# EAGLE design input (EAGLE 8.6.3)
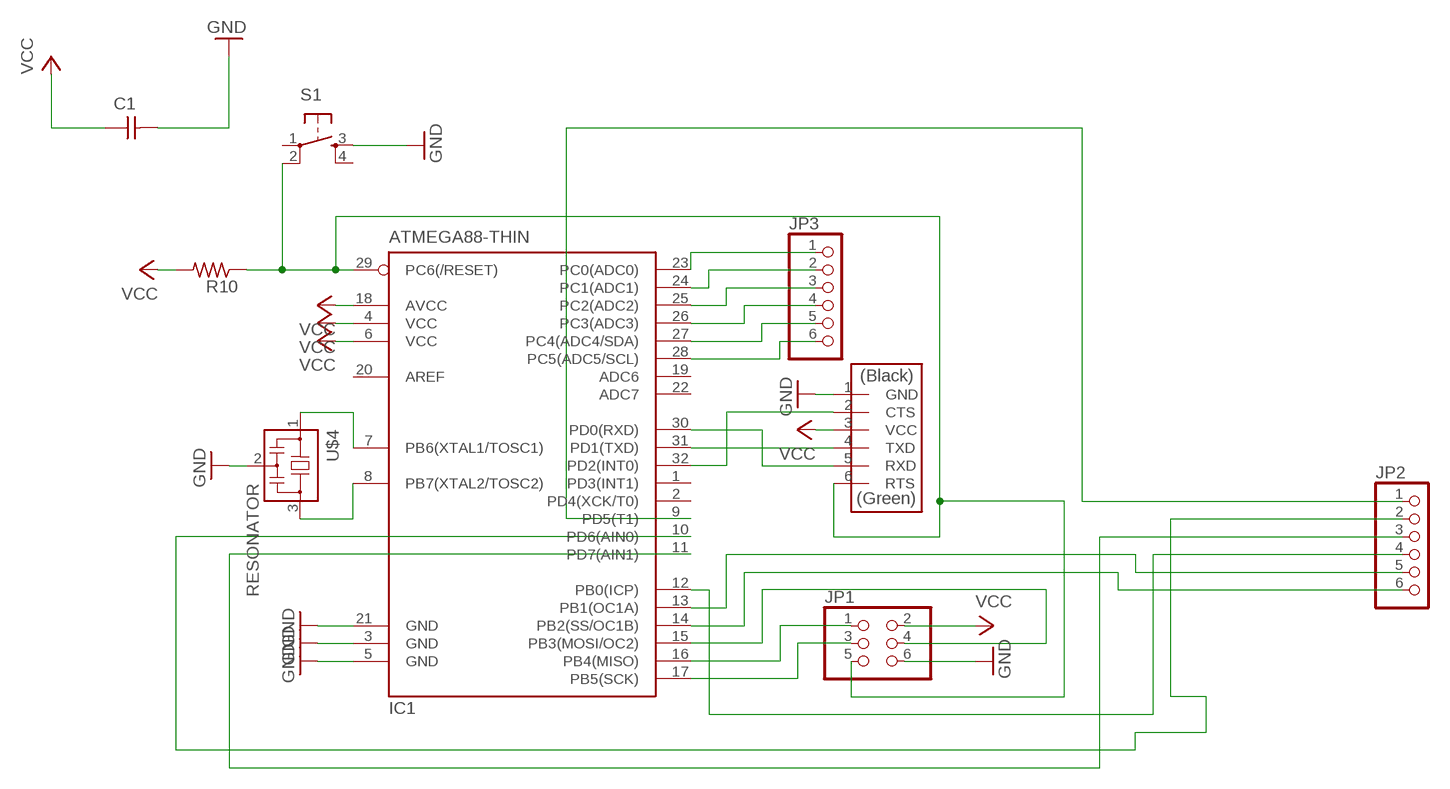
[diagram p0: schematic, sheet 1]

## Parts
C1  CAP-UNPOLARIZEDFAB  [C1206FAB]
IC1  ATMEGA88-THIN  [TQFP32-08THIN]
JP1  PINHD-2X3-SMD  [2X03SMD]
JP2  PINHD-1X6  [1X06]
JP3  PINHD-1X6  [1X06]
R10  RES-US1206FAB  [R1206FAB]
S1  6MM_SWITCH6MM_SWITCH  [6MM_SWITCH]
U$4  RESONATOR  [EFOBM]
U$5  FTDI-SMD-HEADER  [1X06SMD]

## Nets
GND: C1.2 IC1.3(GND) IC1.5(GND) IC1.21(GND) JP1.6 S1.3(S) U$4.2 U$5.1(GND)
N$1: IC1.7(PB6(XTAL1/TOSC1)) U$4.1
N$2: IC1.8(PB7(XTAL2/TOSC2)) U$4.3
N$3: IC1.29(PC6(/RESET)) JP1.5 R10.1 S1.2(P1) U$5.6(RTS)
N$4: IC1.15(PB3(MOSI/OC2)) JP1.4
N$5: IC1.31(PD1(TXD)) U$5.4(TXD)
N$6: IC1.16(PB4(MISO)) JP1.1
N$7: IC1.28(PC5(ADC5/SCL)) JP3.6
N$8: IC1.17(PB5(SCK)) JP1.3
N$9: IC1.30(PD0(RXD)) U$5.5(RXD)
N$10: IC1.32(PD2(INT0)) U$5.2(CTS)
N$11: IC1.27(PC4(ADC4/SDA)) JP3.5
N$12: IC1.26(PC3(ADC3)) JP3.4
N$13: IC1.25(PC2(ADC2)) JP3.3
N$14: IC1.24(PC1(ADC1)) JP3.2
N$15: IC1.23(PC0(ADC0)) JP3.1
N$16: IC1.14(PB2(SS/OC1B)) JP2.6
N$17: IC1.13(PB1(OC1A)) JP2.5
N$18: IC1.12(PB0(ICP)) JP2.4
N$19: IC1.11(PD7(AIN1)) JP2.3
N$20: IC1.10(PD6(AIN0)) JP2.2
N$21: IC1.9(PD5(T1)) JP2.1
VCC: C1.1 IC1.4(VCC) IC1.6(VCC) IC1.18(AVCC) JP1.2 R10.2 U$5.3(VCC)
Unconnected: IC1.1(PD3(INT1)) IC1.2(PD4(XCK/T0)) IC1.19(ADC6) IC1.20(AREF) IC1.22(ADC7) S1.1(P) S1.4(S1)

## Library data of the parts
C1 = fab:CAP-UNPOLARIZED
IC1 = fab:ATMEGA88-THIN
JP1 = fab:PINHD-2X3-SMD: PIN HEADER
JP2 JP3 = adafruit:PINHD-1X6: PIN HEADER
R10 = fab:RES-US: Resistor (US Symbol)
S1 = fab:6MM_SWITCH: OMRON SWITCH
U$4 = fab:RESONATOR
U$5 = fab:FTDI-SMD-HEADER

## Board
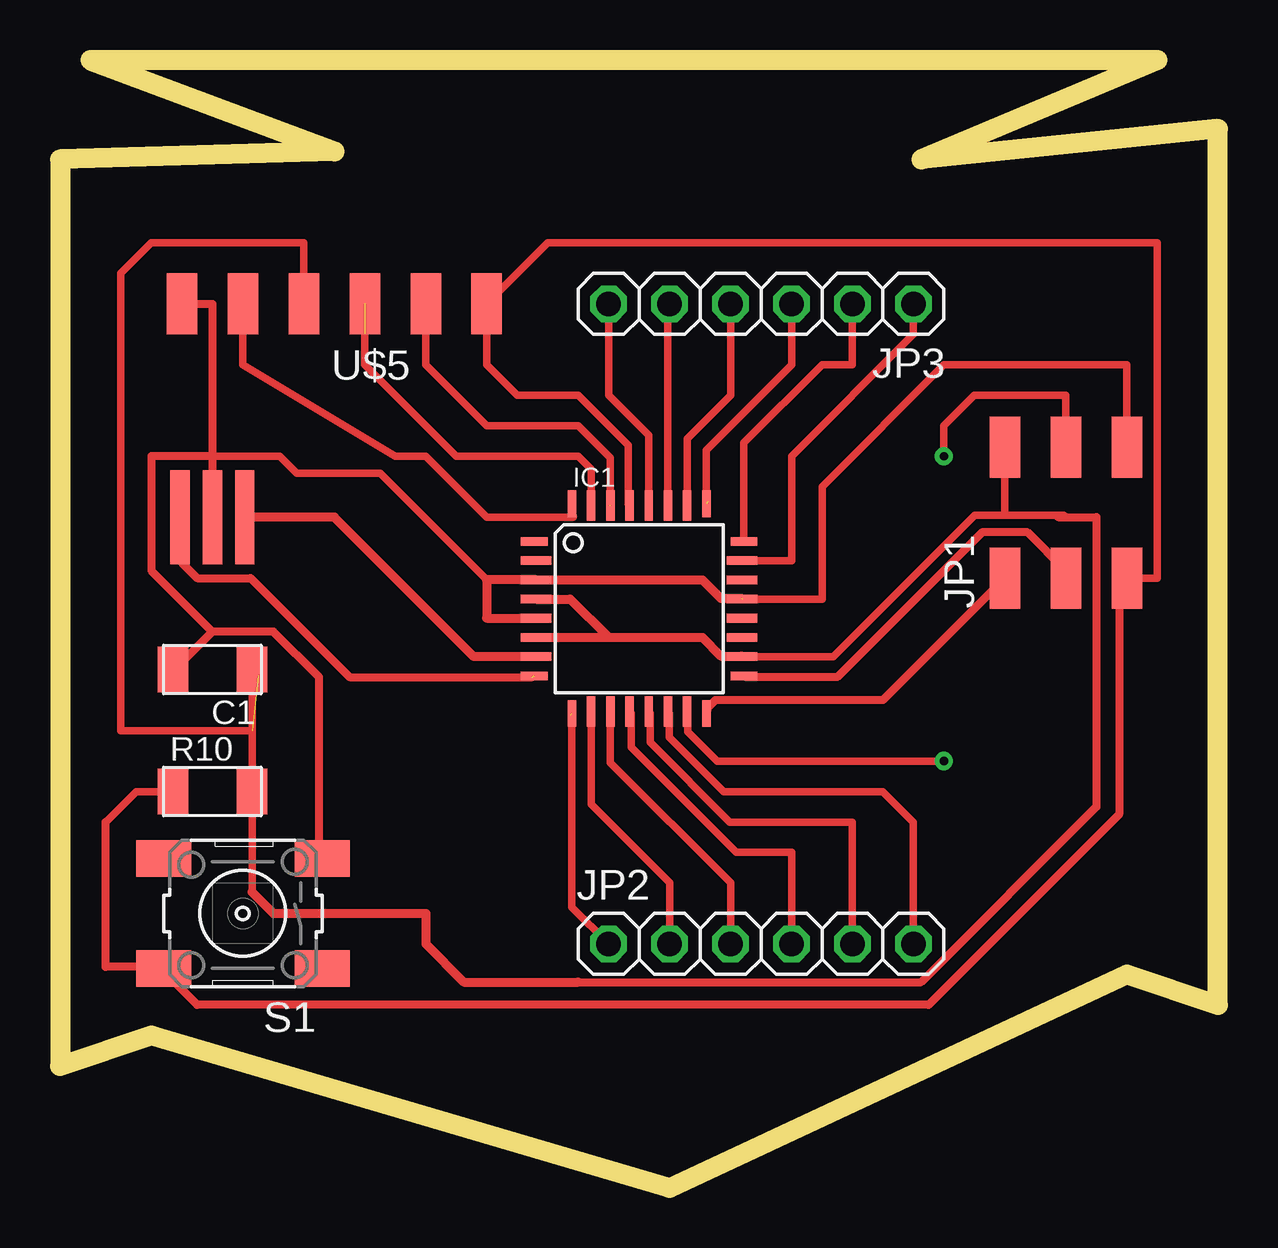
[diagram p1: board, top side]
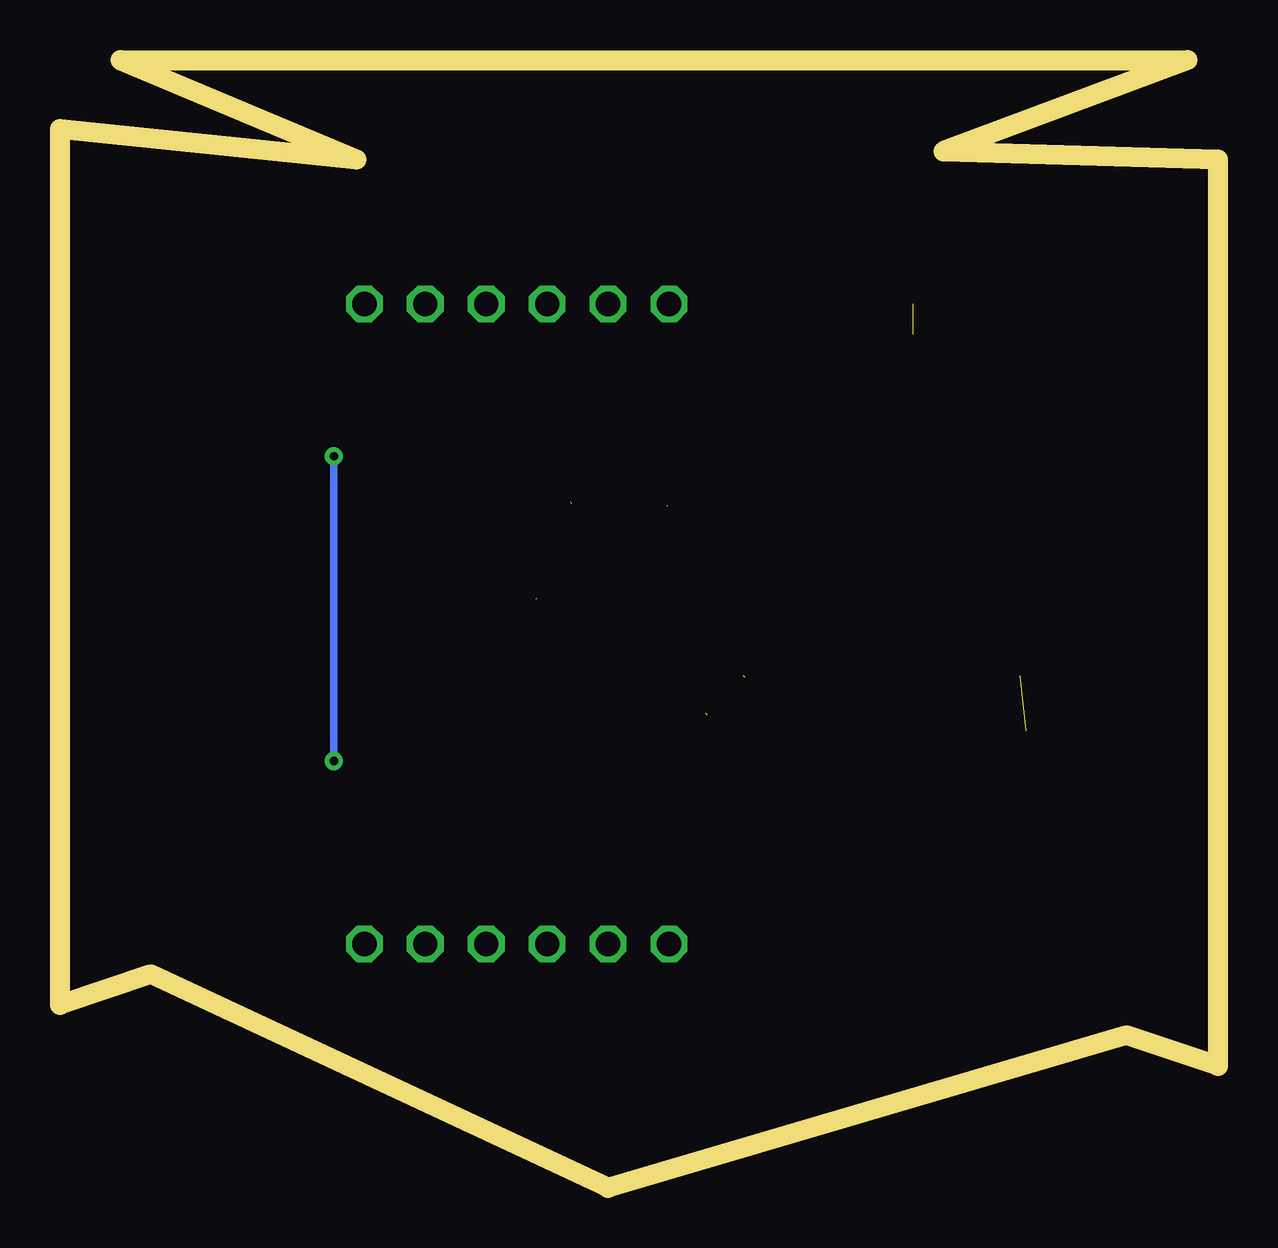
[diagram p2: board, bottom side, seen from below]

Size 48.24 x 46.99 mm. Coordinates in mm from the lower left corner, seen from the top.
Outline: 0,5.08 3.81,6.35 25.4,0 44.45,8.89 48.24,7.62 48.24,44.12 35.89,42.85 45.72,46.99 1.27,46.99 11.43,43.18 0,42.85 0,5.08
Copper layers (1*16): Top 0.035mm / dielectric 1.5mm / Bottom 0.035mm
Design rules "default *": minimum track width 13mil, minimum drill 0.35mm, track to track 16mil, track to pad 16mil, pad to pad 16mil, via to via 16mil, smd to smd 16mil, copper to edge 40mil, drill to drill 6mil, minimum pad ring 10mil, minimum via ring 8mil, stop-mask expansion 4mil, vias tented up to drill 0mil, thermal gap 10mil

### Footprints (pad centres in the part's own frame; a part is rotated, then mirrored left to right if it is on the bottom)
C1206FAB = smd 1.27 x 1.905: 1 -1.651,0; 2 1.651,0
TQFP32-08THIN = smd 1.118 x 0.356: 1 -4.369,2.8; 8 -4.369,-2.8; 17 4.369,-2.8; 24 4.369,2.8 | smd 1.27 x 0.356: 2 -4.293,2; 3 -4.293,1.2; 4 -4.293,0.4; 5 -4.293,-0.4; 6 -4.293,-1.2; 7 -4.293,-2; 18 4.293,-2; 19 4.293,-1.2; 20 4.293,-0.4; 21 4.293,0.4; 22 4.293,1.2; 23 4.293,2 | smd 0.356 x 1.118: 9 -2.8,-4.369; 16 2.8,-4.369; 25 2.8,4.369; 32 -2.8,4.369 | smd 0.356 x 1.27: 10 -2,-4.293; 14 1.2,-4.293; 15 2,-4.293; 26 2,4.293; 27 1.2,4.293; 31 -2,4.293 | smd 0.35 x 1.27: 11 -1.2,-4.293; 12 -0.4,-4.293; 13 0.4,-4.293; 28 0.4,4.293; 29 -0.4,4.293; 30 -1.2,4.293
2X03SMD = smd 2.54 x 1.27: 1 -2.54,2.54; 2 2.92,2.54; 3 -2.54,0; 4 2.92,0; 5 -2.54,-2.54; 6 2.92,-2.54
1X06 = drill 1.016 octagon: 1 -6.35,0; 2 -3.81,0; 3 -1.27,0; 4 1.27,0; 5 3.81,0; 6 6.35,0
R1206FAB = smd 1.27 x 1.905: 1 -1.651,0; 2 1.651,0
6MM_SWITCH = smd 2.286 x 1.524: 1 -3.302,2.286; 2 3.302,2.286; 3 -3.302,-2.286; 4 3.302,-2.286
EFOBM = smd 0.8 x 3.9: 1 -1.35,0; 2 0,0; 3 1.35,0
1X06SMD = smd 2.54 x 1.27: 1 0,6.35; 2 0,3.81; 3 0,1.27; 4 0,-1.27; 5 0,-3.81; 6 0,-6.35

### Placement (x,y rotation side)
C1  6.35,21.59 180 top
IC1  24.13,24.13 0 top
JP1  41.91,27.94 90 top
JP2  29.21,10.16 0 top
JP3  29.21,36.83 180 top
R10  6.35,16.51 0 top
S1  7.62,11.43 180 top
U$4  6.35,27.94 180 top
U$5  11.43,36.83 90 top

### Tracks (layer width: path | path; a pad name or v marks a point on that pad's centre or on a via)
GND  (1 unrouted)
  Top 0.305: 17.78,25.33 13.34,29.77 9.87,29.77 9.15,30.48 6.35,30.48 | IC1.21 31.75,24.53 31.75,29.21 36.83,34.29 44.45,34.29 JP1.6
  Top 0.33: 6.35,23.18 4.76,21.59 C1.2 | 6.35,23.18 8.89,23.18 10.8,21.27 10.8,13.97 S1.3 | 5.08,37.15 U$5.1 6.35,36.83 6.35,30.48 | 6.35,30.48 U$4.2 | 6.35,23.18 3.81,25.72 3.81,30.48 6.35,30.48
  Top 0.381: IC1.5 17.78,23.73 17.78,25.33 IC1.3 26.77,25.33 27.54,24.55 28.4,24.55
  Top 0.457: 4.6,21.43 C1.2 | 5.24,36.99 U$5.1
N$1
  Top 0.381: IC1.7 17.24,22.13 11.43,27.94 U$4.1
N$2  (1 unrouted)
  Top 0.33: 19.69,21.27 12.06,21.27 7.94,25.4 5.72,25.4 5.08,26.04 5.08,27.94 U$4.3
N$3
  Top 0.305: IC1.29 23.68,28.47 23.68,30.93 21.59,33.02 19.05,33.02 17.78,34.29 U$5.6 20.32,39.37 45.72,39.37 45.72,25.4 44.13,25.4 | 1.91,15.24 3.17,16.51 R10.1
  Top 0.33: 1.91,15.24 1.91,9.21 4.13,9.21 S1.2 4.45,8.89 5.72,7.62 36.19,7.62 44.13,15.56 44.13,25.4 JP1.5 44.13,25.72 | 18.1,37.46 U$5.6
  Top 0.381: 17.78,37.15 17.94,37.31
  Top 0.457: 17.78,37.15 U$5.6 17.94,37.31 | 44.29,25.56 JP1.5
N$4  (via drill 0.35)
  Top 0.305: IC1.15 26.16,19.81 26.16,19.01 27.38,17.78 v36.83,17.78 | v36.83,30.48 36.83,31.75 38.1,33.02 41.91,33.02 JP1.4
  Top 0.381: 41.91,31.75 JP1.4
  Bottom 0.305: v36.83,17.78 v36.83,30.48
N$5  (1 unrouted)
  Top 0.305: IC1.31 22.13,29.94 21.59,30.48 16.51,30.48 12.7,34.29 12.7,35.56
N$6
  Top 0.33: JP1.1 34.29,20.32 27.3,20.32 26.99,20 IC1.16
N$7
  Top 0.305: IC1.28 24.53,31.35 22.86,33.02 JP3.6
N$8
  Top 0.33: 41.91,25.72 40.32,27.3 38.42,27.3 32.39,21.27 28.58,21.27 IC1.17
  Top 0.457: 41.91,25.72 JP1.3
N$9  (1 unrouted)
  Top 0.305: U$5.5 15.24,34.29 17.78,31.75 21.59,31.75 22.93,30.41 IC1.30
  Top 0.406: 15.24,36.11 U$5.5
N$10
  Top 0.305: U$5.2 7.62,34.29 13.97,30.48 15.24,30.48 17.78,27.94 21.39,27.94 IC1.32
  Top 0.33: U$5.2 7.62,36.2
  Top 0.457: 7.62,37.15 U$5.2
N$11
  Top 0.305: IC1.27 25.33,36.76 JP3.5
N$12
  Top 0.305: IC1.26 26.13,31.21 27.94,33.02 JP3.4
N$13  (1 unrouted)
  Top 0.305: IC1.25 26.93,30.74 30.48,34.29 JP3.3
N$14
  Top 0.305: IC1.24 28.5,31.04 31.75,34.29 33.02,34.29 JP3.2
N$15
  Top 0.305: IC1.23 30.48,26.13 30.48,27.94 | JP3.1 35.56,35.56 30.48,30.48 30.48,27.94 | 30.48,27.94
N$16
  Top 0.305: IC1.14 25.39,19.77 25.39,18.77 27.65,16.51 34.29,16.51 35.56,15.24 JP2.6
N$17
  Top 0.305: IC1.13 24.59,19.77 24.59,18.56 27.91,15.24 33.02,15.24 JP2.5
N$18
  Top 0.305: IC1.12 23.8,19.77 23.8,18.35 28.18,13.97 30.48,13.97 JP2.4
N$19
  Top 0.305: IC1.11 22.93,17.71 27.94,12.7 JP2.3
N$20
  Top 0.305: IC1.10 22.13,15.97 25.4,12.7 JP2.2
N$21  (1 unrouted)
  Top 0.305: IC1.9 21.33,11.69 JP2.1
VCC  (1 unrouted)
  Top 0.305: IC1.18 32.22,22.13 38.12,28.03 39.37,28.03 | 39.37,28.03 39.37,30.16 39.21,30.32 | 41.91,27.94 41.82,28.03 39.37,28.03 | 8,12.32 R10.2 C1.1 | 8,19.05 2.54,19.05 2.54,38.1 3.81,39.37 10.16,39.37 U$5.3
  Top 0.33: 8.26,21.59 C1.1 | 21.59,8.57 35.88,8.57 43.18,15.88 43.18,27.94 41.91,27.94 41.59,27.94 | 39.21,30.32 39.05,30.48 JP1.2
  Top 0.381: JP1.2 38.99,30.48 | IC1.6 22.86,22.93 | 22.86,22.93 26.77,22.93 27.54,22.15 28.4,22.15 IC1.18 | IC1.4 21.26,24.53 22.86,22.93 | C1.1 8.26,21.34 | 8,12.32 8.89,11.43 15.24,11.43 15.24,10.16 16.83,8.57 21.59,8.57
  Top 0.457: 8.1,21.59 C1.1 8.26,21.75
